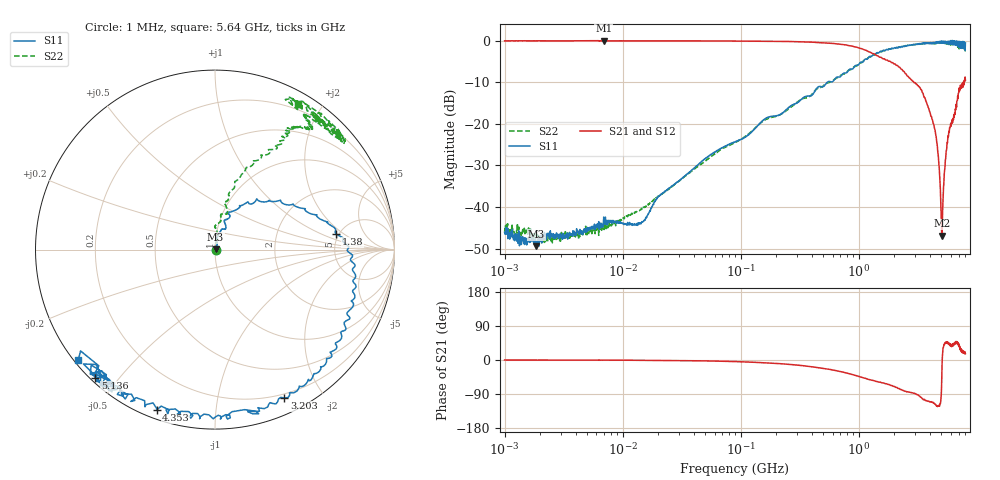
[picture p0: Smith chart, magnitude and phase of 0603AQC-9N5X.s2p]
!s-Parameter Generated by FASTRON Sdn. Bhd.
!FASTRON P/N : 0603AQC-9N5X
!Keysight Technologies: E5071C_MY46733604_B.14.02
!Date: Thu Jun 25 13:51:11 2026
!Version  :Rev00  Thu Jun 25 13:51:11 2026
!Data & Calibration Information:
!Freq  S11:SOLT2(ON)  S21:SOLT2(ON)  S12:SOLT2(ON)  S22:SOLT2(ON)
!PortZ  Port1:50+j0  Port2:50+j0
!When reading reference impedance value at option line is always used.
! Remarks : This data is being provided solely for informational purposes.
# Hz S dB R 50
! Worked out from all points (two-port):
!   1601 points, 1 MHz to 8 GHz, reference 50 ohm
!   highest |S21| = 0.01 dB at 6.912 MHz (marker M1); lowest = -46.9 dB at 5.052 GHz (marker M2)
!   |S21| within 3 dB of the highest: start of sweep to 1.284 GHz
!   lowest |S11| = -49.4 dB at 1.85 MHz (marker M3), VSWR 1.01, Z = 50.3 + j0.0963 ohm
!   |S11| at or under -10 dB: start of sweep to 540.3 MHz
!   |S22| runs from -48.6 to -0.3 dB; largest |S21 - S12| = 0.025
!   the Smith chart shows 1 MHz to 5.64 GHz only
!   S11 on the Smith chart (normalised r, x): 1 MHz: 1.01, -0.00; 1.38 GHz: 4.73, +1.54; 3.203 GHz: 0.16, -1.56; 4.353 GHz: 0.04, -0.70; 5.136 GHz: 0.01, -0.43; 5.64 GHz: 0.01, -0.35
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1000000  -46.10 -0.9  -0.05 -0.1  -0.04 -0.1  -46.00 6.3
1850129  -49.40 16.4  -0.04 -0.2  -0.05 -0.1  -46.80 4.9
4479405  -45.70 30.3  -0.05 -0.3  -0.05 -0.2  -46.40 36.1
6911657  -42.40 21.5  0.01 -0.4  0.00 -0.4  -42.90 33.7
1.406113e7  -44.00 53.1  -0.04 -0.7  -0.06 -0.8  -40.70 56.5
2.00676e7  -37.50 55.8  -0.06 -1.0  -0.06 -1.0  -37.40 74.7
8.994653e7  -24.30 81.8  -0.09 -4.3  -0.09 -4.2  -24.50 76.9
4.006501e8  -13.10 70.0  -0.35 -17.9  -0.36 -17.9  -12.90 71.9
8.377436e8  -6.85 37.2  -1.23 -36.4  -1.23 -36.4  -7.04 70.6
1.380485e9  -3.35 7.4  -3.40 -56.2  -3.42 -56.3  -3.21 58.1
1.7949e9  -2.07 -9.5  -4.95 -64.6  -4.98 -64.8  -2.03 58.0
2.398863e9  -1.30 -35.1  -7.37 -80.6  -7.40 -80.7  -1.36 52.7
3.203473e9  -0.80 -64.9  -10.90 -93.3  -10.90 -93.3  -0.86 56.1
4.352635e9  -0.42 -110.0  -20.70 -115.0  -20.70 -115.0  -0.65 51.0
4.632554e9  -0.37 -123.0  -25.50 -123.0  -25.50 -123.0  -0.67 41.0
4.912472e9  -0.55 -129.0  -35.90 -115.0  -35.90 -115.0  -0.63 42.3
5.052431e9  -0.08 -130.0  -46.90 -40.7  -47.00 -41.8  -0.39 43.9
5.136407e9  -0.20 -133.0  -40.60 19.1  -40.50 19.2  -0.45 46.7
5.64026e9  -0.16 -141.0  -24.60 45.2  -24.50 45.0  -0.60 60.3
6.110812e9  -0.34 -158.0  -19.80 34.9  -19.80 34.6  -0.82 49.7
6.766244e9  -1.14 -150.0  -14.60 48.7  -14.60 48.2  -1.10 82.3
8e9  -0.53 158.0  -9.51 16.5  -9.54 15.8  -1.45 70.2
